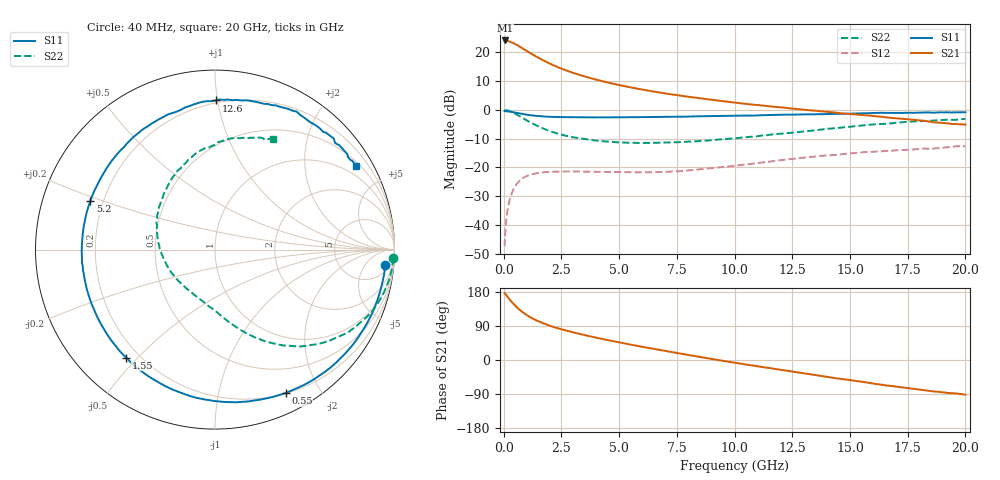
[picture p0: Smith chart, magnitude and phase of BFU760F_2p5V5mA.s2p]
! Filename:  P:\Prog\Test\Noise\ATS_data\Testdata_Net\Split files Spar\BFU760F_2W_C1_Bias1_2.5V_5mA_30mA_D.s2p
! Date/Time: Mon 06/Feb/2012 15:07:55
! BFU760_2W_C1_Bias1_2.5V_5mA_30mA_R.s2p
! MDIF S-parameter v. bias file
! BFU760_2W_C1_2.5V_5mA_30mA
! Date/time Fri Mar 18 11:16:19 2011
! bias mode 1
! bias variable = I_out
! VAR bias_var= 1
! VAR V_out= 2.5000
! VAR I_out= 4.9650
! VAR V_in= 0.7554
! VAR I_in= 0.0129
! Device data file deembeded for feedlines and parallel
! Original file: \Split files Spar\BFU760_2W_C1_Bias1_2.5V_5mA_30mA_R.s2p
! Feed-files: PR003V01_101208_Feed1.s2p, PR003V01_101208_Feed2.s2p
! Parallel-file: PR003V01_101208_Par.s2p
# MHz S MA R 50
!  Freq-MHz  S11-mag  S11-arg  S21-mag  S21-arg  S12-mag  S12-arg  S22-mag  S22-arg
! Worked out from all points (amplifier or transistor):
!   167 points, 40 MHz to 20 GHz, reference 50 ohm
!   highest |S21| = 24.1 dB at 50 MHz (marker M1)
!   |S21| within 3 dB of that: start of sweep to 862.7 MHz
!   unconditionally stable (mu >= 1): 6.003 GHz to 12.65 GHz
!   at 550 MHz: K = 0.07, MSG = 24.3 dB, |S12| = -25.9 dB
!   at 4.2 GHz: K = 0.68, MSG = 15.8 dB, |S12| = -21.5 dB
!   at 20 GHz: K = 0.77, MSG = 3.8 dB, |S12| = -12.6 dB
!   S11 on the Smith chart (normalised r, x): 40 MHz: 10, -17; 550 MHz: 0.20, -1.59; 1.55 GHz: 0.15, -0.46; 5.2 GHz: 0.15, +0.18; 12.6 GHz: 0.18, +0.99; 20 GHz: 0.64, +3.54
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40  0.9526 -5.0  16.09 176.9  0.004295 81.6  0.9942 -2.8
50  0.9484 -6.3  16.11 175.6  0.005912 82.3  0.9934 -3.6
60  0.9523 -7.3  15.89 174.9  0.006513 81.4  0.9936 -4.2
80  0.9512 -9.9  16.04 173.6  0.008652 82.4  0.9917 -5.7
140  0.9476 -17.4  15.87 168.8  0.01508 79.5  0.9838 -10.0
280  0.9332 -34.4  15.28 158.1  0.02925 71.0  0.9489 -19.6
420  0.9117 -50.4  14.53 148.4  0.04152 62.6  0.8963 -28.3
550  0.8909 -63.8  13.63 140.3  0.05077 55.5  0.8375 -35.6
800  0.8512 -86.1  11.88 127.1  0.06411 44.4  0.734 -47.0
1050  0.8193 -103.8  10.26 116.6  0.07229 36.0  0.6402 -55.9
1300  0.7966 -118.0  8.945 108.0  0.07757 29.7  0.5661 -62.7
1550  0.7798 -129.5  7.866 100.9  0.08089 24.7  0.5071 -68.4
1900  0.7637 -142.4  6.668 92.5  0.08349 19.3  0.4437 -75.2
2250  0.7529 -152.6  5.743 85.5  0.08489 15.3  0.398 -80.8
3400  0.7426 -176.2  3.931 67.2  0.08517 7.2  0.317 -96.5
5200  0.7456 158.7  2.601 44.1  0.0828 3.3  0.2716 -120.9
6800  0.7565 141.3  1.993 26.0  0.08347 4.7  0.2695 -143.2
10200  0.7961 109.9  1.315 -9.1  0.1093 7.0  0.3277 167.7
12600  0.8311 89.6  1.045 -31.7  0.1424 -0.3  0.4069 137.3
13400  0.8377 83.5  0.9756 -38.8  0.1542 -4.8  0.4386 127.5
16800  0.8877 56.1  0.7254 -68.6  0.1958 -25.6  0.5843 89.8
20000  0.9127 30.6  0.5576 -91.6  0.2337 -48.7  0.6982 62.2
